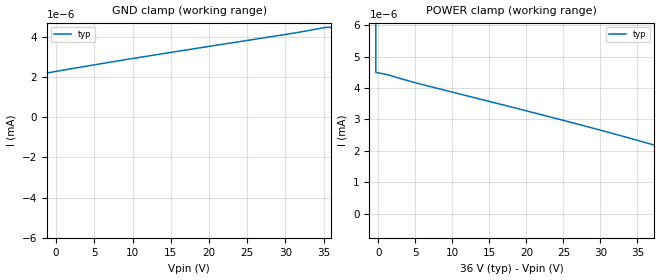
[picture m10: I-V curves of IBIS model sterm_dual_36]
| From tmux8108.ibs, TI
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| sterm_dual_36
[Model]   sterm_dual_36
Model_type   Terminator
|   typ   min   max
C_comp   4.014581e-12   NA   NA
[Voltage Range]   36   NA   NA
[Temperature Range]   27   NA   NA
[Power Clamp Reference]   36   NA   NA
[GND Clamp Reference]   0   NA   NA
[GND Clamp]
|   Voltage   I(typ)   I(min)   I(max)
-41V      -1.145A    NA         NA
-36.33V   -6.477nA   NA         NA
-35.56V   -524.1pA   NA         NA
-30.89V   -218.2pA   NA         NA
-16.89V   1.024nA    NA         NA
-4.444V   1.967nA    NA         NA
9.556V    2.881nA    NA         NA
35.22V    4.455nA    NA         NA
36V       4.464nA    NA         NA
[POWER Clamp]
|   Voltage   I(typ)   I(min)   I(max)
-5V       744mA      NA         NA
-1.111V   26.13mA    NA         NA
-333.3mV  4.496nA    NA         NA
1.222V    4.424nA    NA         NA
5.111V    4.16nA     NA         NA
26.89V    2.853nA    NA         NA
40.89V    1.936nA    NA         NA
52.56V    1.052nA    NA         NA
66.56V    -191.2pA   NA         NA
68.89V    -365.1pA   NA         NA
72V       -549pA     NA         NA
